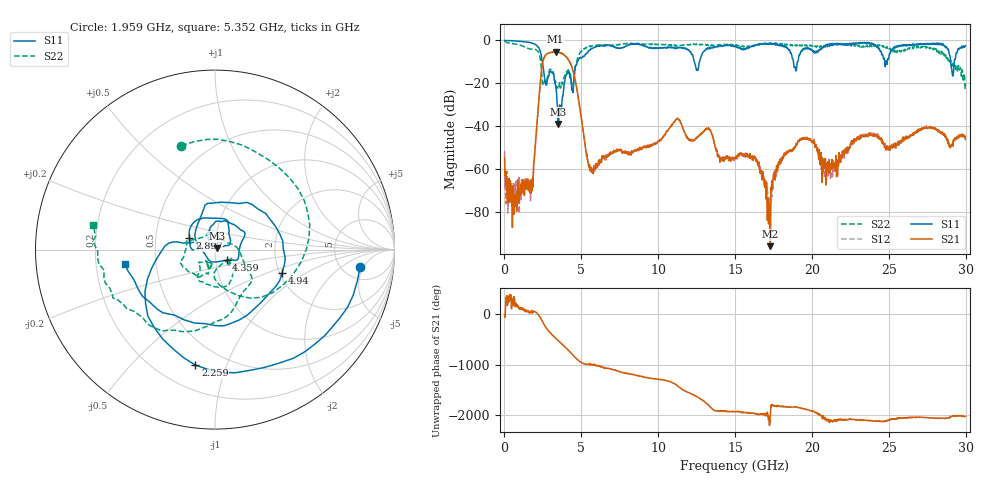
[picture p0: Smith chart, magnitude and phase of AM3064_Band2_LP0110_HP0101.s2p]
# Hz S DB R 50.0
!freq dBS11 angS11 dBS21 angS21 dBS12 angS12 dBS22 angS22
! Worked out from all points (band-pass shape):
!   1600 points, 10 MHz to 29.98 GHz, reference 50 ohm
!   highest |S21| = -5.26 dB at 3.328 GHz (marker M1); lowest = -95.7 dB at 17.29 GHz (marker M2)
!   |S21| within 3 dB of the highest: 2.568 GHz to 4.082 GHz (1.514 GHz wide, 45.5 % of centre)
!   lowest |S11| = -38.9 dB at 3.478 GHz (marker M3), VSWR 1.02, Z = 50.9 + j0.658 ohm
!   |S11| at or under -10 dB: 2.454 GHz to 4.733 GHz (2.279 GHz wide, 63.4 % of centre); 12.36 GHz to 12.68 GHz (319.8 MHz wide, 2.56 % of centre); 18.8 GHz to 19.05 GHz (252.9 MHz wide, 1.34 % of centre)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
!   |S22| runs from -23.5 to -0.3 dB; largest |S21 - S12| = 0.02
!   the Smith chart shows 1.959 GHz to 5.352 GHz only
!   S11 on the Smith chart (normalised r, x): 1.959 GHz: 7.26, -4.23; 2.259 GHz: 0.35, -0.78; 2.897 GHz: 0.74, +0.10; 4.359 GHz: 1.13, -0.14; 4.94 GHz: 2.06, -0.63; 5.352 GHz: 0.33, -0.07
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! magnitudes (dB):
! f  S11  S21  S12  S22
! 10 MHz  0.0  -54.6  -51.5  -0.3
! 666 MHz  -0.3  -74.7  -71.2  -1.6
! 1.697 GHz  -1.1  -65.0  -74.9  -4.0
! 1.959 GHz  -1.8  -53.0  -53.2  -4.3
! 2.259 GHz  -3.7  -25.7  -25.6  -6.3
! 2.897 GHz  -16.1  -5.8  -5.8  -14.3
! 3.328 GHz  -21.0  -5.3  -5.3  -19.3
! 3.478 GHz  -38.9  -5.4  -5.4  -22.1
! 4.359 GHz  -21.1  -11.8  -11.7  -20.0
! 4.94 GHz  -8.1  -33.3  -33.3  -5.3
! 5.015 GHz  -8.2  -36.9  -36.8  -5.1
! 5.352 GHz  -5.9  -54.1  -53.3  -3.2
! 10 GHz  -3.6  -46.8  -47.1  -1.9
! 11.27 GHz  -3.4  -36.4  -36.3  -2.5
! 15 GHz  -2.7  -54.7  -55.1  -2.0
! 16.32 GHz  -2.2  -55.1  -54.3  -2.2
! 17.29 GHz  -1.7  -95.7  -80.0  -1.4
! 18.1 GHz  -2.5  -54.2  -55.4  -1.5
! 19.99 GHz  -4.4  -47.0  -46.8  -2.3
! 21.08 GHz  -2.4  -61.5  -58.4  -2.2
! 25 GHz  -8.1  -49.7  -50.5  -3.2
! 29.98 GHz  -2.5  -46.1  -44.8  -20.3
